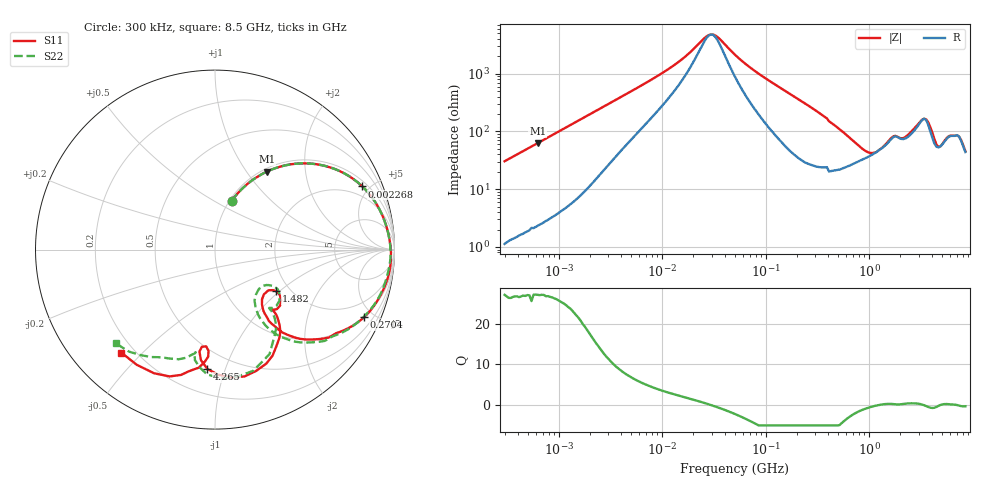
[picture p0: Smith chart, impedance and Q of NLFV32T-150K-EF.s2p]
! S-parameter Generated by TDK Corporation
! Copyright(C) 2015 TDK Corporation.
! All Rights Reserved.
! TDK P/N: NLFV32T-150K-EF (Inductors)
! Property: L=15uH at 2.52MHz
! Size(LxWxT): 3.2x2.5x2.2mm, 0.126x0.098x0.087inches
! Model Type: s2p (Touchstone File Format Version 1.0)
! Frequency: DC=Yes Start=0.3MHz Stop=8500MHz 225points Log-sweep
! Note:
! Model Generated on Jun. 23, 2015
! Hash(MD5):
! Port Assignments:
!  1 ---@@@--- 2
! Applicable Conditions:
!  Temperature = 25 degC
!  DC Bias Current = 0 A
!  Small Signal Operation
! Terms and conditions regarding TDK Simulation Models
! (1)This simulation model is being provided solely for informational purposes. Please refer to the specifications of the products in terms of detailed characteristics of such products.
! (2)In no event shall TDK Corporation of any of its subsidiaries be liable for any loss or damage arising, directly or indirectly,
!  From any information contained in this simulation model, including, but not limited to loss or damages arising from any inaccuracies, omissions or errors in connection with such information.
! (3)Any and all copyrights on this simulation model are owned by TDK Corporation.
!  Duplication or redistribution of this simulation model without prior written permission from TDK Corporation is prohibited.
! (4)This simulation model is subject to any modification or change without any prior notice.
! (5)Neither TDK Corporation nor any of its subsidiaries shall make any warranty, express or implied,
!  Including but not limited to the correctness, implied warranties of merchantability and fitness for a particular purpose with respect to this simulation models.
! (6)The use of this simulation model shall be deemed to have consented to the terms and conditions hereof.
# MHz S MA R 50
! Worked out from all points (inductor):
!   224 points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, 300 kHz to 8.5 GHz, reference 50 ohm
!   read as one part in series: L = 16.1 uH near 314.1 kHz
!   highest Q = 27.1 at 626 kHz (marker M1), where L = 15.9 uH
!   self-resonance near 29.67 MHz
!   S11 on the Smith chart (normalised r, x): 300 kHz: 1.02, +0.61; 2.268 MHz: 1.30, +4.51; 270.4 MHz: 0.98, -4.42; 1.482 GHz: 1.70, -0.95; 4.265 GHz: 0.36, -0.87; 8.5 GHz: 0.15, -0.43
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0.3  0.2873 71.2  0.9451 -16.7  0.9506 -16.9  0.2857 71.2
0.6259918  0.5222 56.3  0.8341 -31.5  0.836 -31.8  0.5218 56.4
1.72111  0.8452 29.5  0.4945 -57.6  0.4954 -57.9  0.8458 29.4
2.267783  0.893 23.2  0.3966 -63.1  0.3976 -63.4  0.8939 23.1
9.430415  0.9696 5.4  0.1008 -69.8  0.1008 -70.1  0.9696 5.2
28.42509  0.98 -0.4  0.02083 -9.2  0.02084 -9.6  0.9788 -0.6
34.1636  0.9807 -1.2  0.02257 26.4  0.02258 26.1  0.9791 -1.5
51.67171  0.9816 -3.5  0.04775 62.8  0.04778 62.5  0.9779 -3.8
270.4017  0.9122 -24.4  0.3343 59.4  0.3345 59.1  0.9012 -25.6
283.1228  0.9042 -25.5  0.3495 58.1  0.3496 57.8  0.8935 -26.8
491.5417  0.732 -43.2  0.5701 35.8  0.5702 35.3  0.7213 -45.9
778.4218  0.4983 -52.9  0.6831 10.3  0.6828 10.0  0.4796 -56.6
1124.446  0.374 -44.3  0.678 -11.1  0.6773 -11.3  0.3386 -47.6
1481.602  0.4112 -34.3  0.598 -26.8  0.5986 -27.4  0.3596 -33.4
1551.304  0.4296 -34.5  0.5746 -28.8  0.5751 -29.6  0.3828 -31.8
2346.313  0.4843 -46.5  0.5095 -44.1  0.5095 -44.2  0.4621 -47.3
3091.568  0.6374 -57.5  0.3465 -55.7  0.3465 -55.9  0.622 -59.4
3548.748  0.714 -71.4  0.288 -43.1  0.2887 -43.7  0.7083 -72.6
4265.177  0.6665 -93.6  0.4101 -37.3  0.4098 -37.3  0.6972 -93.6
5126.239  0.5412 -95.2  0.4423 -63.7  0.4415 -64.1  0.5817 -100.7
6754.475  0.6958 -102.4  0.2942 -79.7  0.2946 -80.1  0.6713 -116.7
8500  0.7758 -132.3  0.2615 -77.4  0.2608 -76.6  0.7595 -136.6
